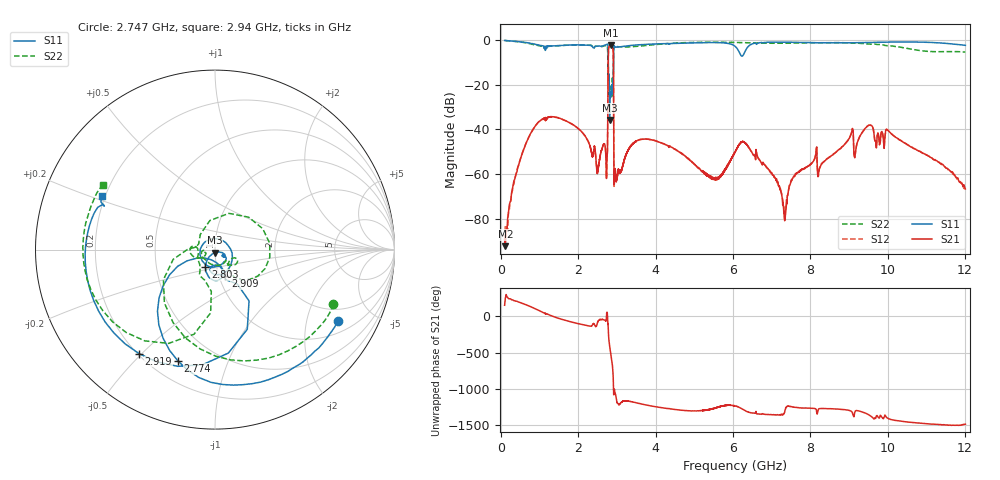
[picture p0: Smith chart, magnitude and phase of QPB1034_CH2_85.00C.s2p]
! TDS: k:\Engsetup\Winsaw\QPB1034_ALL
! Channel 1
! Ports=1 2
! seg 1=100.000000 1100.000000 51
! seg 2=1101.000000 1301.000000 201
! seg 3=1302.000000 2302.000000 101
! seg 4=2303.000000 3503.000000 1201
! seg 5=3504.000000 5204.000000 171
! seg 6=5205.000000 6405.000000 1201
! seg 7=6406.000000 8506.000000 211
! seg 8=8507.000000 12007.000000 176
! Points=3313
! FailCode=0
! Topology=ALL_SE(12)
!VNA Cal loaded =QPB1034_ALL_85C
!PS1(V)= 5.000
!PS(mA)= 0.449
!PS2(V)= 0.630
!PS(mA)= -0.003
!PS3(V)= 1.170
!PS(mA)= 0.000
!PS4(V)= 0.630
!PS(mA)= -0.003
!Temp (C)= 85.00
# MHz S DB R 50
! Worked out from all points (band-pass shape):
!   3313 points, 100 MHz to 12.01 GHz, reference 50 ohm
!   highest |S21| = -2.37 dB at 2.84 GHz (marker M1); lowest = -92.1 dB at 120 MHz (marker M2)
!   |S21| within 3 dB of the highest: 2.783 GHz to 2.908 GHz (125.1 MHz wide, 4.4 % of centre)
!   lowest |S11| = -35.7 dB at 2.812 GHz (marker M3), VSWR 1.03, Z = 49.8 - j1.62 ohm
!   |S11| at or under -10 dB: 2.781 GHz to 2.913 GHz (132.3 MHz wide, 4.65 % of centre)
!   |S22| runs from -25.4 to -0.3 dB; largest |S21 - S12| = 0.0043
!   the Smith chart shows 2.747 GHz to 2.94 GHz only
!   S11 on the Smith chart (normalised r, x): 2.747 GHz: 1.46, -3.10; 2.774 GHz: 0.31, -0.67; 2.803 GHz: 0.88, -0.17; 2.909 GHz: 1.07, -0.33; 2.919 GHz: 0.21, -0.49; 2.94 GHz: 0.19, +0.22
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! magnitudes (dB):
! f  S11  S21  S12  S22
! 100 MHz  -0.3  -89.5  -89.4  -0.3
! 120 MHz  -0.4  -92.1  -82.7  -0.4
! 240 MHz  -0.5  -72.5  -72.6  -0.5
! 500 MHz  -0.9  -53.8  -53.6  -1.0
! 1.1 GHz  -2.8  -35.2  -35.2  -3.0
! 2.434 GHz  -3.0  -48.5  -48.5  -3.0
! 2.494 GHz  -2.9  -59.1  -59.1  -2.9
! 2.747 GHz  -2.0  -52.3  -52.1  -2.8
! 2.774 GHz  -3.7  -14.6  -14.6  -13.3
! 2.803 GHz  -19.2  -2.9  -2.9  -18.5
! 2.812 GHz  -35.7  -2.6  -2.6  -21.3
! 2.84 GHz  -25.8  -2.4  -2.4  -22.0
! 2.896 GHz  -18.1  -3.7  -3.7  -20.7
! 2.909 GHz  -16.0  -5.9  -5.9  -15.9
! 2.919 GHz  -2.9  -39.1  -39.1  -3.0
! 2.94 GHz  -3.1  -59.0  -58.8  -2.9
! 3.754 GHz  -2.0  -44.3  -44.4  -2.6
! 5.406 GHz  -1.3  -61.1  -61.0  -1.1
! 6.268 GHz  -6.8  -45.6  -45.6  -1.3
! 7.336 GHz  -1.1  -80.8  -80.6  -1.6
! 9.707 GHz  -1.2  -48.3  -48.4  -2.1
! 12.01 GHz  -2.5  -66.6  -66.5  -5.5
